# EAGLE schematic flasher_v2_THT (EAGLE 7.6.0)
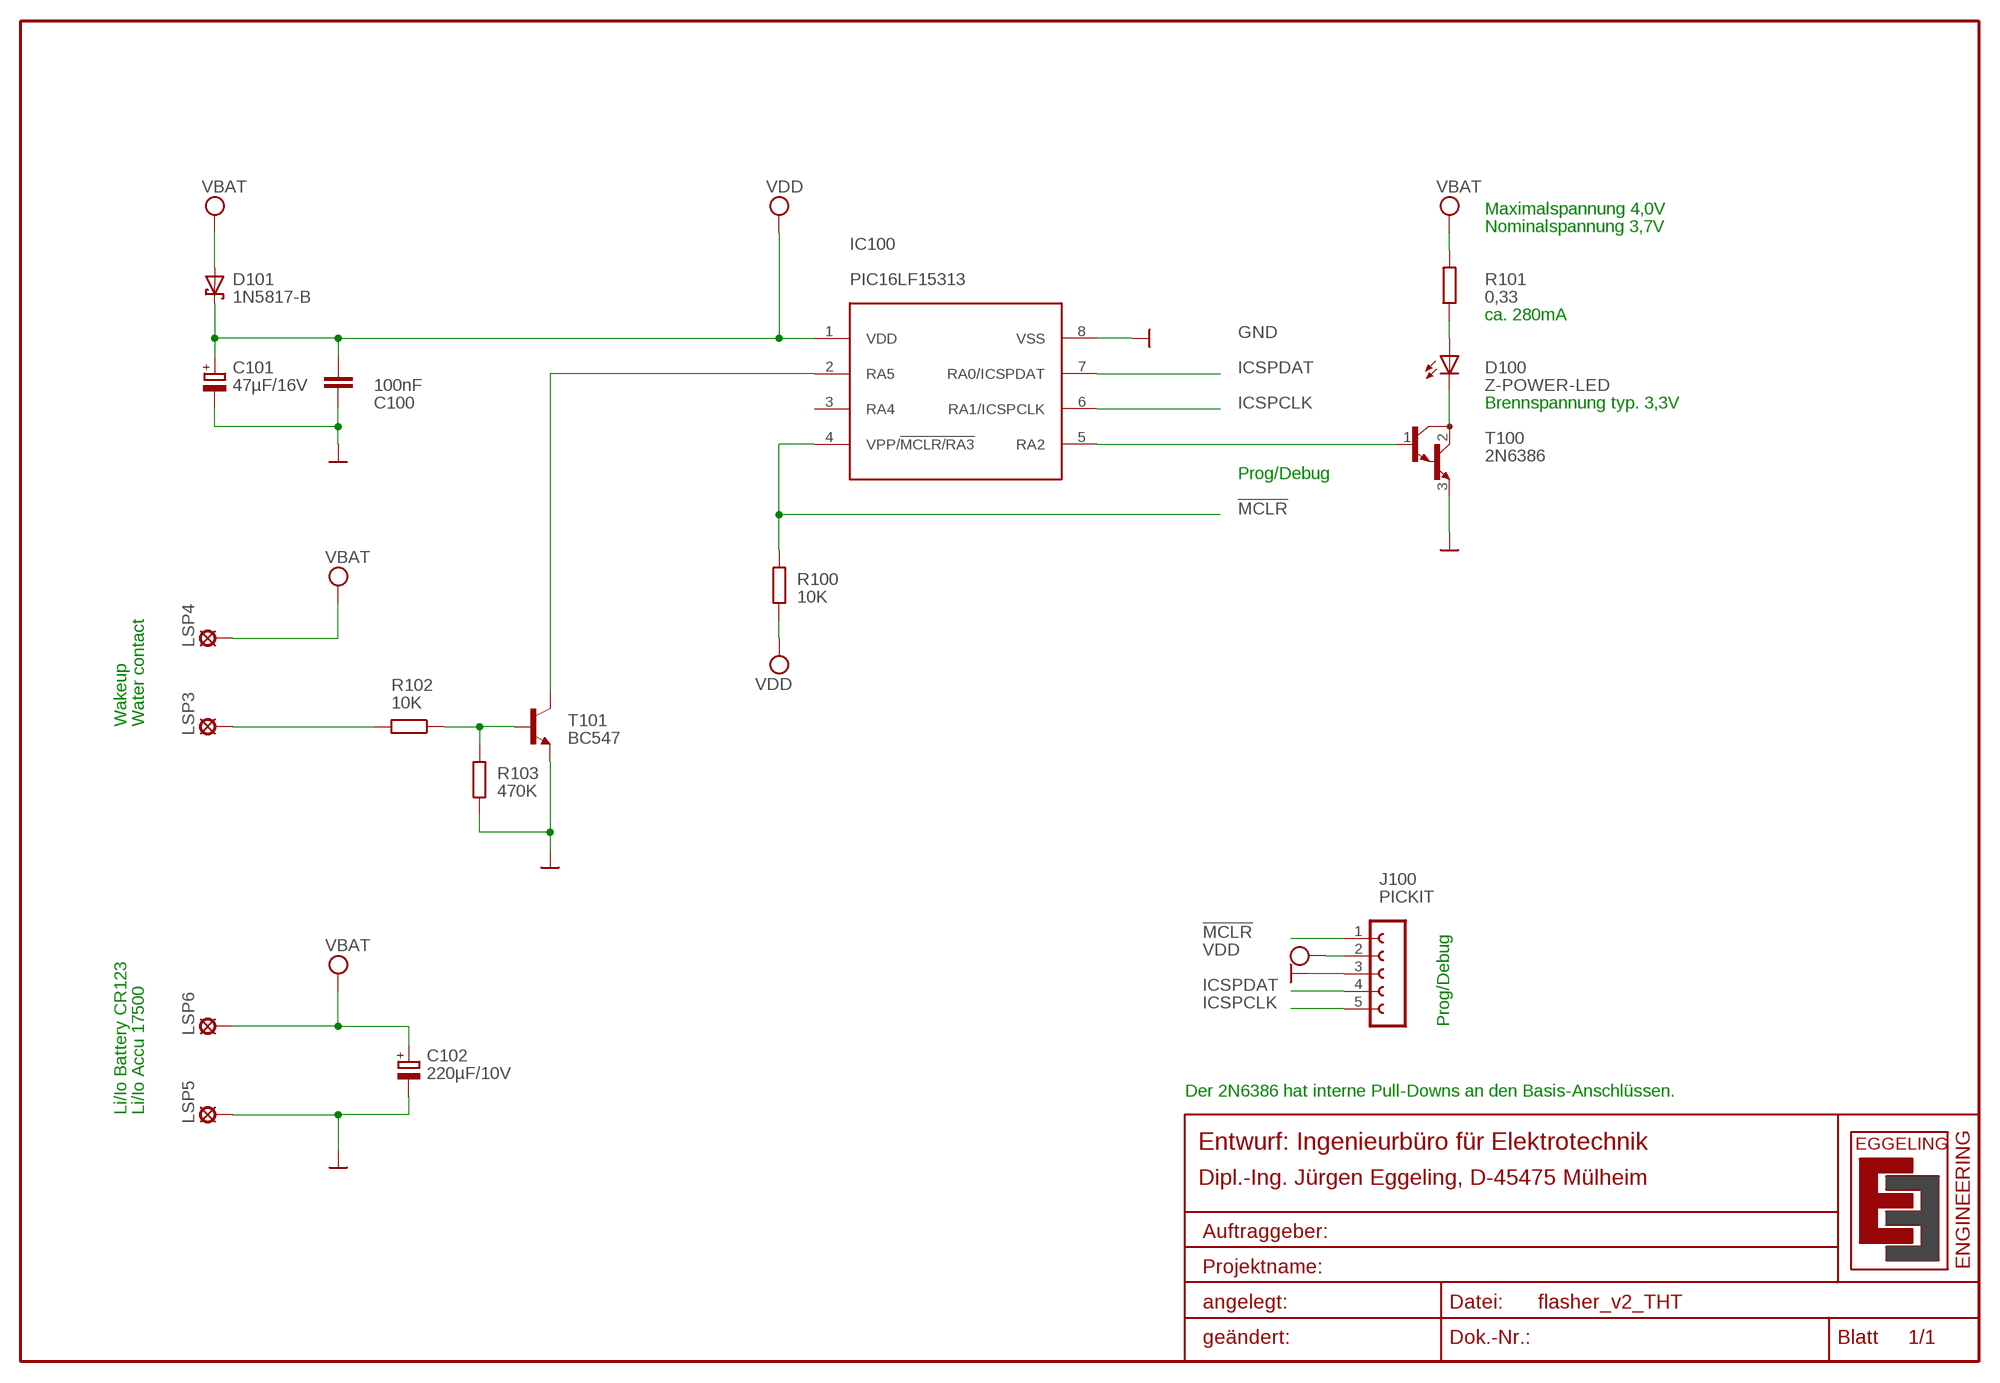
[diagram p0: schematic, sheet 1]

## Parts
C100  100nF  C-EUC0805  [C0805]
C101  47µF/16V  CPOL-EUE2,5-6E  [E2,5-6E]
C102  220µF/10V  CPOL-EUE5-10.5  [E5-10,5]
D100  Z-POWER-LED  [Z-POWER-LED-PCB-TYPE]
D101  1N5817-B  [DO41-7.6]
IC100  PIC16LF15313  [DIL8]
J100  PICKIT  FE05-1  [FE05-1]
LSP3  LSP10  [LSP10]
LSP4  LSP10  [LSP10]
LSP5  LSP10  [LSP10]
LSP6  LSP10  [LSP10]
R100  10K  R-EU_R0805  [R0805]
R101  0,33  R-EU_R0805  [R0805]
R102  10K  R-EU_R0805  [R0805]
R103  470K  R-EU_R0805  [R0805]
T100  2N6386  BU807  [TO220]
T101  BC547  [TO92]

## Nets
!MCLR: IC100.4(VPP/!MCLR/RA3) J100.1 R100.2
EN_PWR2: LSP3.MP R102.2
GND: C100.2 C101.- C102.- IC100.8(VSS) J100.3 LSP5.MP R103.2 T100.3(E) T101.1(E)
ICSPCLK: IC100.6(RA1/ICSPCLK) J100.5
ICSPDAT: IC100.7(RA0/ICSPDAT) J100.4
INPUT: IC100.5(RA2) T100.1(B)
LED_K: D100.C T100.2(C)
N$1: D100.A R101.1
N$2: R102.1 R103.1 T101.2(B)
N$3: IC100.2(RA5) T101.3(C)
VCC: C102.+ D101.A LSP4.MP LSP6.MP R101.2 ; supply symbol labelled VBAT
VDD: C100.1 C101.+ D101.C IC100.1(VDD) J100.2 R100.1
Unconnected: IC100.3(RA4)

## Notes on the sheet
- Maximalspannung 4,0V
- Nominalspannung 3,7V
- ca. 280mA
- Brennspannung typ. 3,3V
- Prog/Debug
- Wakeup | Water contact
- Prog/Debug
- Der 2N6386 hat interne Pull-Downs an den Basis-Anschlüssen.
- Li/Io Battery CR123 | Li/Io Accu 17500

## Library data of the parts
C100 = rcl:C-EU: CAPACITOR, European symbol
C101 C102 = rcl:CPOL-EU: POLARIZED CAPACITOR, European symbol
D100 = led:Z-POWER-LED: Z-Power LED
D101 = diode:1N581*: 1.0A SCHOTTKY BARRIER RECTIFIER
IC100 = flasher_pcb:PIC16LF15313
J100 = con-lsta:FE05-1: FEMALE HEADER; OC_FARNELL: unknown; OC_NEWARK: unknown
LSP3-LSP6 = solpad:LSP10: SOLDER PAD
R100-R103 = rcl:R-EU_: RESISTOR, European symbol
T100 = transistor:BU807: NPN BIPOLAR DARLINGTON TRANSISTOR
T101 = transistor:BC547: NPN TRANSISTOR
